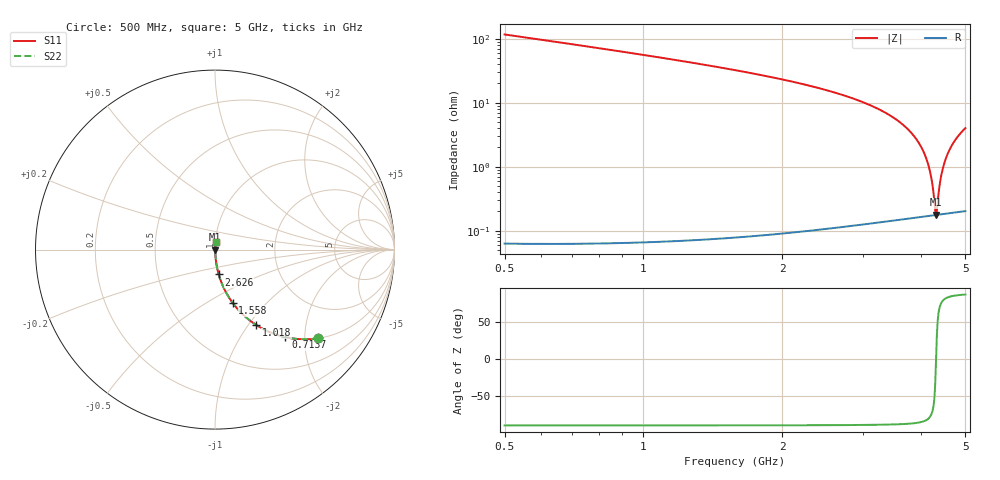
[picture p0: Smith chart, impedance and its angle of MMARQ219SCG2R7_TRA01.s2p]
! MMARQ219SCG2R7_TRA01  S-PARAMETER MODEL  ( General Type )
! Model Generated by TAIYO YUDEN Corporation (http://www.ty-top.com)
! Version 1.0
! TAIYO YUDEN Control No. 160201
! Copyright(c) 2016 TAIYO YUDEN CO.,LTD. All Rights Reserved.
! Product Description (link to TY-COMPAS)
! https://ds.yuden.co.jp/TYCOMPAS/or/detail?pn=MMARQ219SCG2R7BTRA01&u=M
! Products Name : Multilayer Ceramic Capacitors
! Characteristics :
!  Capacitance : 2.7 pF , Rated Voltage : 250V , TCC : CG / C0G
!  Case Size : 2.0 x 1.25 / 0.079 x 0.049 [mm/inch] , Thickness : 0.85 / 0.033 [mm/inch]
!  (Conditions: Temperature = 25 degC , DC Bias Current/Voltage = 0A / 0V)
! External Node Assignments :
!  1  o---| |---o  2
! GND o---------o GND
! Frequency Range : 500MHz  -  5000MHz  [ 401 STEP ]
# MHz S RI R 50
! Freq[MHz].  S11 Real  S11 Imag  S21 Real  S21 Imag  S12 Real  S12 Imag  S22 Real  S22 Imag
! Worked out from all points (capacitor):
!   401 points, 500 MHz to 5 GHz, reference 50 ohm
!   read as one part in series: C = 2.7 pF near 522.5 MHz
!   lowest |Z| = 179 mohm at 4.314 GHz (marker M1)
!   series resonance near 4.319 GHz, so ESL is about 500 pH
!   S11 on the Smith chart (normalised r, x): 500 MHz: 1.00, -2.33; 713.8 MHz: 1.00, -1.61; 1.018 GHz: 1.00, -1.09; 1.558 GHz: 1.00, -0.66; 2.626 GHz: 1.00, -0.28; 5 GHz: 1.00, +0.08
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500  0.5751 -0.4941  0.4249 0.4941  0.4249 0.4941  0.5751 -0.4941
713.75  0.3924 -0.4879  0.6076 0.4879  0.6076 0.4879  0.3924 -0.4879
1017.5  0.2307 -0.4207  0.7693 0.4207  0.7693 0.4207  0.2307 -0.4207
1253.75  0.1568 -0.3628  0.8432 0.3628  0.8432 0.3628  0.1568 -0.3628
1557.5  0.0983 -0.2966  0.9017 0.2966  0.9017 0.2966  0.0983 -0.2966
2007.5  0.051 -0.2181  0.949 0.2181  0.949 0.2181  0.051 -0.2181
2626.25  0.0206 -0.1382  0.9794 0.1382  0.9794 0.1382  0.0206 -0.1382
2750  0.017 -0.1249  0.983 0.1249  0.983 0.1249  0.017 -0.1249
3503.75  0.00471 -0.057  0.9953 0.057  0.9953 0.057  0.00471 -0.057
3807.5  0.00274 -0.0342  0.9973 0.0342  0.9973 0.0342  0.00274 -0.0342
4021.25  0.00202 -0.0194  0.998 0.0194  0.998 0.0194  0.00202 -0.0194
4167.5  0.00179 -0.00966  0.9982 0.00966  0.9982 0.00966  0.00179 -0.00966
4212.5  0.00176 -0.00674  0.9982 0.00674  0.9982 0.00674  0.00176 -0.00674
4257.5  0.00175 -0.00386  0.9983 0.00386  0.9983 0.00386  0.00175 -0.00386
4291.25  0.00175 -0.00172  0.9982 0.00172  0.9982 0.00172  0.00175 -0.00172
4313.75  0.00176 -0.000301  0.9982 0.000301  0.9982 0.000301  0.00176 -0.000301
4336.25  0.00177 0.00111  0.9982 -0.00111  0.9982 -0.00111  0.00177 0.00111
4392.5  0.00181 0.0046  0.9982 -0.0046  0.9982 -0.0046  0.00181 0.0046
4426.25  0.00185 0.00668  0.9982 -0.00668  0.9982 -0.00668  0.00185 0.00668
4538.75  0.00203 0.0135  0.998 -0.0135  0.998 -0.0135  0.00203 0.0135
4730  0.00253 0.0247  0.9975 -0.0247  0.9975 -0.0247  0.00253 0.0247
5000  0.00361 0.0398  0.9964 -0.0398  0.9964 -0.0398  0.00361 0.0398
